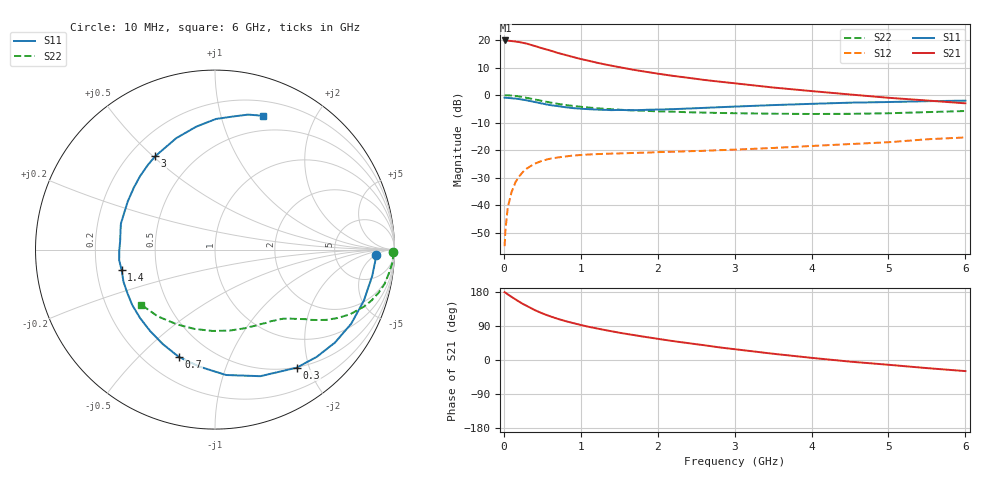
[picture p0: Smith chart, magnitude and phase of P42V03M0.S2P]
! SIEMENS Small Signal Semiconductors
! BFP182
! Si NPN RF Bipolar Junction Transistor in SOT143
! VCE = 2 V  IC = 3 mA
! Common Emitter S-Parameters:  March  1996
# GHz  S  MA  R  50
!  f  S11  S21  S12  S22
! GHz  MAG  ANG  MAG  ANG  MAG  ANG  MAG  ANG
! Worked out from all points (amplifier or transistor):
!   36 points, 10 MHz to 6 GHz, reference 50 ohm
!   highest |S21| = 19.8 dB at 20 MHz (marker M1)
!   |S21| within 3 dB of that: start of sweep to 518.3 MHz
!   unconditionally stable (mu >= 1): 1.917 GHz to 5.824 GHz
!   at 250 MHz: K = 0.16, MSG = 23.4 dB, |S12| = -27.9 dB
!   at 1.4 GHz: K = 0.79, MSG = 16.0 dB, |S12| = -21.3 dB
!   at 6 GHz: K = 0.98, MSG = 6.2 dB, |S12| = -15.4 dB
!   S11 on the Smith chart (normalised r, x): 10 MHz: 17, -5; 300 MHz: 0.49, -1.80; 700 MHz: 0.33, -0.66; 1.4 GHz: 0.31, -0.10; 3 GHz: 0.30, +0.51; 6 GHz: 0.34, +1.36
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0.01  0.896 -1.9  9.769 178.9  0.0018 84.5  0.9941 -0.8
0.02  0.8956 -3.9  9.821 177.8  0.0034 82.1  0.9928 -1.6
0.05  0.8882 -9.5  9.757 173.3  0.0089 85.8  0.9922 -3.9
0.1  0.8769 -18.9  9.58 166.7  0.0173 78.5  0.978 -7.7
0.2  0.8455 -37.8  9.184 153.7  0.0334 68.9  0.9425 -14.8
0.25  0.8236 -46.5  8.878 147.7  0.0405 64.7  0.9173 -18.0
0.3  0.8001 -55.3  8.586 142.5  0.0465 60.2  0.8891 -20.9
0.4  0.7491 -70.3  7.811 131.9  0.0567 53.1  0.8344 -25.6
0.5  0.7013 -85.0  7.065 123.0  0.0642 46.9  0.7816 -29.2
0.6  0.6578 -97.6  6.473 115.4  0.0698 41.9  0.7346 -32.2
0.7  0.6308 -108.7  5.833 108.7  0.0736 38.2  0.6946 -34.4
0.8  0.6015 -118.9  5.36 102.7  0.0766 34.9  0.6612 -36.3
0.9  0.58 -128.6  4.918 97.5  0.0798 32.3  0.6352 -37.6
1.1  0.555 -146.1  4.211 87.7  0.0833 28.5  0.5944 -40.5
1.4  0.5327 -167.5  3.418 75.9  0.0865 24.6  0.5532 -44.1
1.8  0.536 169.3  2.714 62.1  0.0898 22.7  0.5199 -49.1
2.2  0.5554 151.0  2.232 49.9  0.0935 21.7  0.4986 -54.9
3  0.6178 122.6  1.638 28.5  0.102 21.6  0.4684 -69.4
3.5  0.6576 109.1  1.372 16.5  0.1095 21.5  0.4585 -79.9
4.5  0.7278 89.6  1.025 -4.3  0.1288 20.5  0.4564 -104.5
5.5  0.7745 76.2  0.797 -21.4  0.1573 17.6  0.49 -130.6
6  0.7921 70.3  0.708 -29.3  0.1701 13.9  0.5132 -143.2
